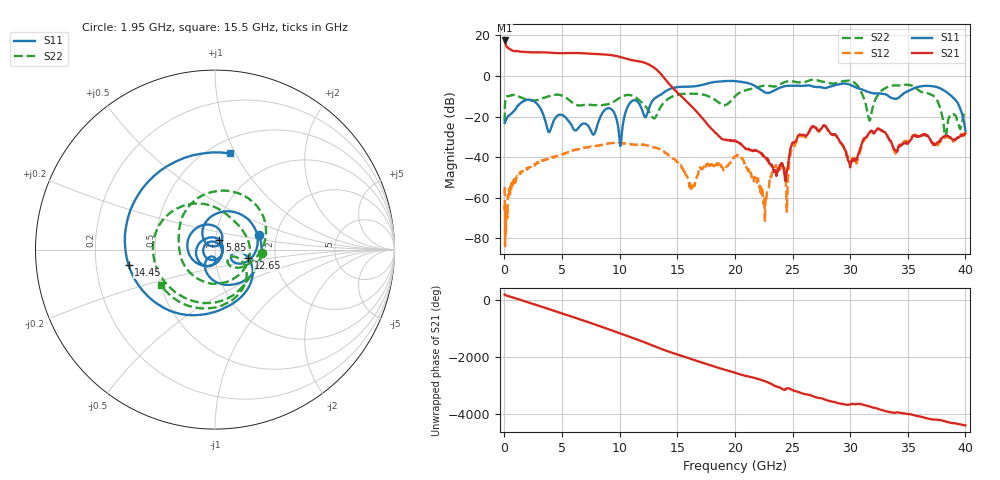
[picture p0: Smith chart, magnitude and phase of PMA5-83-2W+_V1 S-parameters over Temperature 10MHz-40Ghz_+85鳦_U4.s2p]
!Mini-Circuits Laboratory
!S-Parameters
!Model: US-AMP-1
!Run / Lot / Date Code: N/A / N/A / N/A
!Fixture: N/A, Pressing Arm: N/A
!Network Analyzer: NFA N8975A;  Serial number: 74408
!Date: 11/29/2023 at 10:19:47 AM
!No.: Unit# 1 (U4)
!Tested with: +85°C
! 2 port cal with Bias Tee PE1622 in line. No normalization applied. Bias cond 2: Vdd= 12V, Idd= 400mA, Vg2= 5V, starting point for Vg1= -2V
# Hz  S  dB  R  50
!Frequency  S11 dB  S11 Deg  S21 dB  S21 Deg  S12 dB  S12 Deg  S22 dB  S22 Deg
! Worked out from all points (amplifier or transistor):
!   826 points, 10 MHz to 40 GHz, reference 50 ohm
!   highest |S21| = 17.5 dB at 20 MHz (marker M1)
!   |S21| within 3 dB of that: start of sweep to 180.1 MHz
!   unconditionally stable (mu >= 1): start of sweep to end of sweep
!   at 5.6 GHz: K = 9.74, MAG = 11.6 dB, |S12| = -37.7 dB
!   at 19.4 GHz: K = 1293.78, MAG = -27.9 dB, |S12| = -44.2 dB
!   at 40 GHz: K = 319.32, MAG = -28.2 dB, |S12| = -28.0 dB
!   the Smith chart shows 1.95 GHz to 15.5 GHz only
!   S11 on the Smith chart (normalised r, x): 1.95 GHz: 1.61, +0.28; 5.85 GHz: 1.05, +0.11; 12.65 GHz: 1.45, -0.14; 14.45 GHz: 0.35, -0.08; 15.5 GHz: 0.63, +0.95
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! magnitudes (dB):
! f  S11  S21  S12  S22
! 10 MHz  -23.1  17.3  -54.9  -22.4
! 20 MHz  -23.0  17.5  -56.7  -18.7
! 90 MHz  -22.2  15.8  -76.9  -11.1
! 500 MHz  -19.1  13.1  -58.2  -9.7
! 1.95 GHz  -11.8  11.7  -46.2  -11.7
! 5.85 GHz  -24.6  11.3  -37.0  -12.9
! 6.7 GHz  -23.9  11.2  -35.6  -14.5
! 12.65 GHz  -14.3  5.2  -34.7  -18.6
! 13.35 GHz  -9.9  2.3  -35.8  -17.5
! 14.45 GHz  -6.2  -5.0  -40.2  -10.4
! 15.5 GHz  -5.3  -10.8  -45.9  -8.9
! 20.05 GHz  -2.6  -32.1  -39.5  -9.8
! 22.6 GHz  -8.1  -40.1  -72.0  -4.8
! 23.45 GHz  -7.0  -47.5  -44.6  -5.2
! 24.4 GHz  -5.0  -51.9  -50.5  -2.9
! 26.7 GHz  -5.1  -24.9  -25.3  -1.9
! 30 GHz  -4.4  -45.1  -42.4  -2.4
! 31.7 GHz  -8.1  -27.7  -27.9  -22.0
! 33.35 GHz  -10.0  -30.9  -30.8  -5.3
! 37.7 GHz  -5.8  -32.3  -33.3  -14.0
! 38.25 GHz  -7.5  -29.6  -30.4  -29.7
! 40 GHz  -26.9  -28.3  -28.0  -17.2
